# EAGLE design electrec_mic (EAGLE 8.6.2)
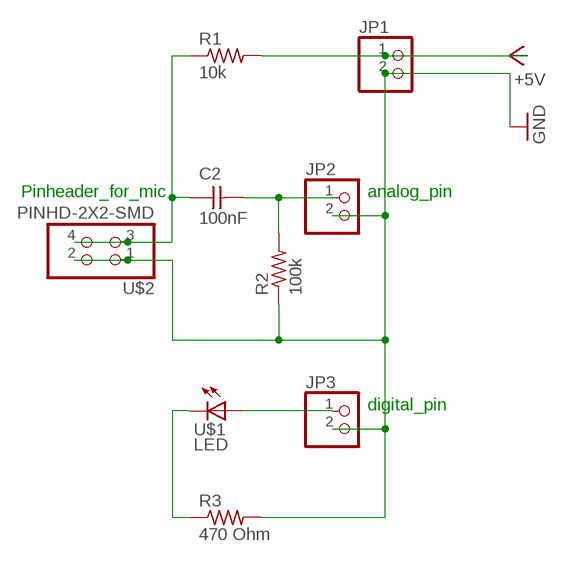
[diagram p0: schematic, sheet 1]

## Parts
C2  100nF  CAP-UNPOLARIZED  [C1206]
JP1  PINHD-1X2/90  [1X02/90]
JP2  PINHD-1X2/90  [1X02/90]
JP3  PINHD-1X2/90  [1X02/90]
R1  10k  RES-US1206  [R1206]
R2  100k  RES-US1206  [R1206]
R3  470 Ohm  RES-US1206  [R1206]
U$1  LED  [LED1206]
U$2  PINHD-2X2-SMD  [2X02SMD]

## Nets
+5V: JP1.1 R1.2
GND: JP1.2 JP2.2 JP3.2 R2.1 R3.2 U$2.1 U$2.2
N$1: JP3.1 U$1.1(A)
N$2: C2.1 R1.1 U$2.3 U$2.4
N$5: C2.2 JP2.1 R2.2
N$6: R3.1 U$1.2(C)

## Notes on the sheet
- Pinheader_for_mic | analog_pin
- digital_pin

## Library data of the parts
C2 = fab:CAP-UNPOLARIZED
JP1-JP3 = pinhead:PINHD-1X2: PIN HEADER
R1-R3 = fab:RES-US: Resistor (US Symbol)
U$1 = fab:LED: LED
U$2 = fab:PINHD-2X2-SMD

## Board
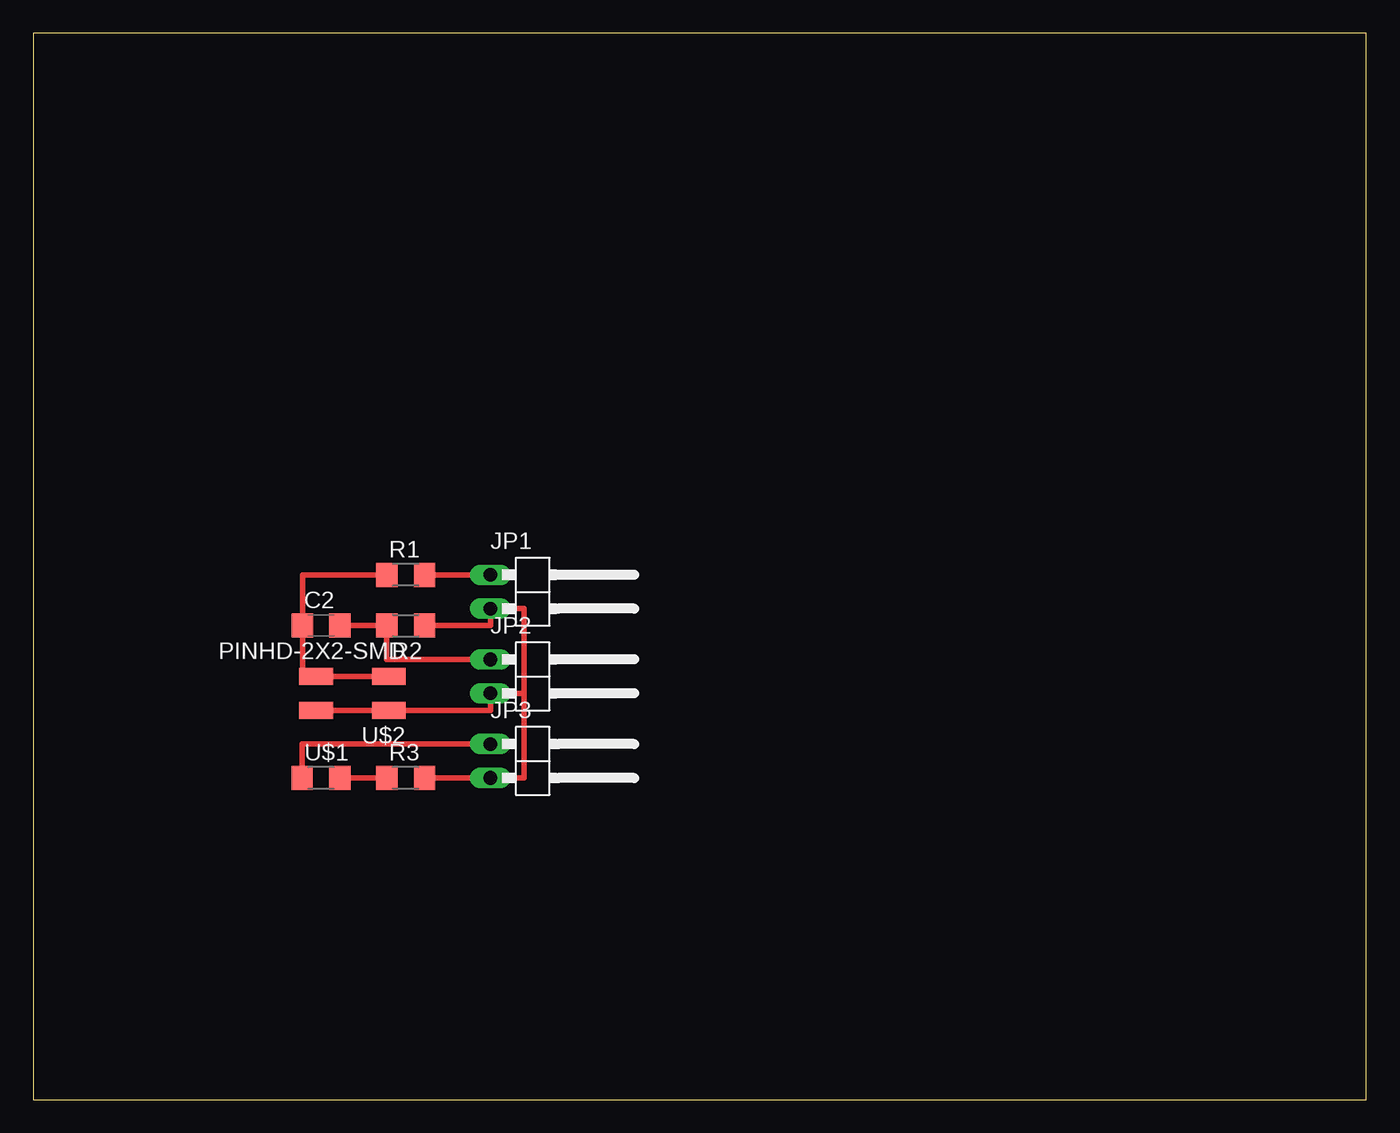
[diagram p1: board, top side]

Size 100 x 80 mm. Coordinates in mm from the lower left corner, seen from the top.
Outline: 0,0 100,0 100,80 0,80 0,0
Copper layers (1*16): Top 0.035mm / dielectric 1.5mm / Bottom 0.035mm
Design rules "fab_mod": minimum track width 10mil, minimum drill 0.4mm, track to track 0.42mm, track to pad 0.42mm, pad to pad 0.42mm, via to via 0.42mm, smd to smd 0.42mm, copper to edge 40mil, drill to drill 6mil, minimum pad ring 10mil, minimum via ring 8mil, stop-mask expansion 4mil, vias tented up to drill 0mil, thermal gap 10mil

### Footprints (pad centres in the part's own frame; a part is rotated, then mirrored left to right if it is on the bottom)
C1206 = smd 1.6 x 1.8: 1 -1.4,0; 2 1.4,0
1X02/90 = drill 1.016 long: 1 -1.27,-3.81; 2 1.27,-3.81
R1206 = smd 1.6 x 1.803: 1 -1.422,0; 2 1.422,0
LED1206 = smd 1.6 x 1.803: 1 -1.422,0; 2 1.422,0
2X02SMD = smd 2.54 x 1.27: 1 -2.54,1.27; 2 2.92,1.27; 3 -2.54,-1.27; 4 2.92,-1.27

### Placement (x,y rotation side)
C2  21.59,35.56 0 top
JP1  38.1,38.1 270 top
JP2  38.1,31.75 270 top
JP3  38.1,25.4 270 top
R1  27.94,39.37 0 top
R2  27.94,35.56 180 top
R3  27.94,24.13 0 top
U$1  21.59,24.13 0 top
U$2  24.13,30.48 180 top

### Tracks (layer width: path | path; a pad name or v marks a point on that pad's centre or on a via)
+5V
  Top 0.406: JP1.1 R1.2
GND
  Top 0.406: 36.83,30.48 36.83,36.83 JP1.2 34.29,35.56 R2.1 | 36.83,30.48 36.83,24.13 JP3.2 R3.2 | U$2.2 U$2.1 34.29,29.21 JP2.2 36.83,30.48
N$1
  Top 0.406: U$1.1 20.17,26.67 JP3.1
N$2
  Top 0.406: R1.1 20.19,39.37 C2.1 20.19,31.75 U$2.4 U$2.3
N$5
  Top 0.406: C2.2 R2.2 26.52,33.02 JP2.1
N$6
  Top 0.406: U$1.2 R3.1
